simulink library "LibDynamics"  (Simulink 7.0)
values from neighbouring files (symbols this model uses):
  delay = ones(nTbl,1) * mean(valveDelay)    [analysis.m]
  dof = [1 2 3 4 5 6]    [initialize.m]    (also in StaticLiftTransform.m = [3 4 5]; accelEnvelope.m = varargin{1}{1}; displEnvelope.m = varargin{1}{1}; displPivotEnvelope.m = varargin{1}{1})
  flowCanon = 63090.2    [initialize.m]
  forceCanon = 0.00444822    [initialize.m]
  gasConstant = 1.8    [initialize.m]
  gee = geeCanon / linAccelCanon * ~isempty(find(dof==3))    [initialize.m]    (also in accelA2T.m = 0; accelEnvelope.m = varargin{1}{6}; accelT2A.m = 0)
  inertia = inertia + inertiaP2Q([0 0 0], massA(i), cgA(:,i)-cg,  									inertiaCanon, massCanon)    [initialize.m]
  inertiaCanon = 2.9264264e-04    (= 0.00029264264)    [initialize.m]
  initDispl = zeros(6, 1)    [initialize.m]
  lengthCanon = 25.4    [initialize.m]
  linAccelCanon = 9810.0    (= 9810)    [initialize.m]    (also in StaticLiftTransform.m; accelJacobian.m = canon(3); accelP2Q.m = canon(3))
  linDisplCanon = 1    [initialize.m]    (also in StaticLiftTransform.m; displJacobian.m = canon(1))
  linVelocCanon = 1000.0    (= 1000)    [initialize.m]    (also in StaticLiftTransform.m)
  mass = ones(3, 1) * (sum(massA) + massT + massS)    [initialize.m]
  massCanon = 0.4535924e-06    (= 4.535924e-07)    [initialize.m]
  maxDispl = max(abs(maxDispl), abs(minDispl))    [initialize.m]    (also in Tutorial.m = 0.4)
  maxVeloc = max(abs(maxVeloc), abs(minVeloc))    [analysis.m]    (also in initialize.m; rampth.m = 2 * maxDispl / (nVeloc * deltaT); Tutorial.m = 1.234)
  modalCG = [0 0 1000]    [initialize.m]
  modalDamp = [4 5 6]    [initialize.m]    (also in resondemo.m = eval(get(findobj(fig, 'Tag', 'modalDamp'), 'String')))
  modalFreq = [7 6 5]    [initialize.m]    (also in resondemo.m = tableFreq * freqRatio)
  modalMass = 0    [initialize.m]    (also in resondemo.m = tableMass * massRatio)
  oilDamping = 2 * damping * 0.01 * 2 * pi .* oilColumn .* massQ * massCanon    [initialize.m]
  oilSpring = bulkModulus * pressCanon  			.* (area1 * areaCanon ./ length1 + area2 * areaCanon ./ length2)    [initialize.m]
  precharge = 2000    [initialize.m]
  pumpFlow = 1e10    (= 10000000000)    [initialize.m]
  rotAccelCanon = pi/180    (= 0.0174532925199)    [initialize.m]    (also in StaticLiftTransform.m; accelJacobian.m = canon(7); accelP2Q.m = canon(7); bodyAccel.m = canon(3))
  rotDisplCanon = pi/180    (= 0.0174532925199)    [initialize.m]    (also in StaticLiftTransform.m; accelA2T.m = canon(5); accelP2Q.m = canon(5); accelT2A.m = canon(5))
  rotForceCanon = 1000    [initialize.m]    (also in StaticLiftTransform.m)
  rotVelocCanon = pi/180    (= 0.0174532925199)    [initialize.m]    (also in StaticLiftTransform.m; accelJacobian.m = canon(6); accelP2Q.m = canon(6); bodyAccel.m = canon(2))
  samplePeriod = controlPeriod/upsampleFactor    (= 0.00048828125)    [initialize.m]    (also in viewer.m = eval(getHeaderValue(header, 'DELTA_T')))
  supplyPress = 3000    [initialize.m]
  vmax = ( (maxFlow' * flowCanon ./ (area1 * areaCanon)) / linVelocCanon)'    [initialize.m]
  volume = 160    [initialize.m]    (also in quake.m = volume / 231.0)
  volumeCanon = 3785412.0    (= 3785412)    [initialize.m]
undefined symbols (not defined in the file or in its folder): drive, drum, friction, gear, motDisplCanon, motor, motTorqueCanon, motVelocCanon, params, yieldDispl
libraries: LibDynamics x26, LibTransforms x12, aerospace x6, simulink x2
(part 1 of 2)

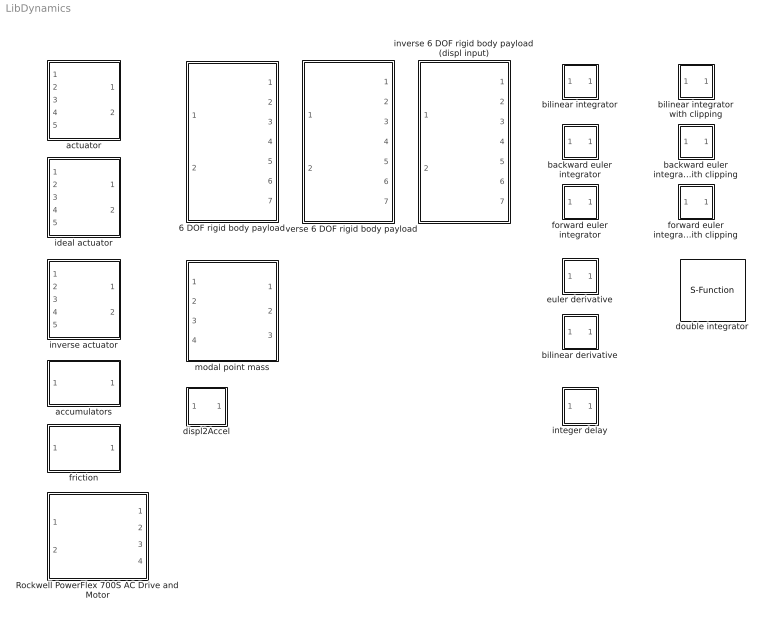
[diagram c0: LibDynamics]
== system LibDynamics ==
  6 DOF rigid body payload : Subsystem  mask(6 DOF Rigid Body Payload Model){mass=mass, inertia=diag(inertia), gee=gee, massCanon=massCanon, inertiaCanon=inertiaCanon, linVelocCanon=linVelocCanon, linAccelCanon=linAccelCanon, rotDisplCanon=rotDisplCanon, rotVelocCanon=rotVelocCanon, rotAccelCanon=rotAccelCanon, rotForceCanon=rotForceCanon, initialPosition=zeros(6,1), samplePeriod=samplePeriod}
      mask prompts: gee "Gravity constant"; massCanon "Canonical mass units"; inertiaCanon "Canonical inertia units"; linVelocCanon "Canonical linear veloc units"; linAccelCanon "Canonical linear accel units"; rotDisplCanon "Canonical rotary displ units"; rotVelocCanon "Canonical rotary veloc units"; rotAccelCanon "Canonical rotary accel units"; rotForceCanon "Canonical rotary force units"; initialPosition "Initial position"; samplePeriod "Sample period (sec)"
      mask init:
      | % invert mass vector
      | invMass = zeros(3,1);
      | nonzero = find(mass>0);
      | invMass(nonzero) = 1 ./ mass(nonzero);
      | 
      | % invert inertia matrix
      | invInertia = zeros(3, 3);
      | nonzero    = find(sum(inertia, 1)>0);
      | invInertia(:,nonzero) = pinv(inertia(nonzero,:));
  Rockwell PowerFlex 700S AC Drive and Motor : Subsystem  mask(Rockwell PowerFlex 700S AC Drive and Motor){MotorNPRPM4=drive.MotorNPRPM4, MotorNPPower5=drive.MotorNPPower5, TotalInertia9=drive.TotalInertia9, SpdTrim3Scale24=drive.SpdTrim3Scale24, InertAccelGain57=drive.InertAccelGain57, SpdRegPGain81=drive.SpdRegPGain81, SpdRegIGain82=drive.SpdRegIGain82, SpdRegAntiBckup84=drive.SpdRegAntiBckup84, SpdErrFiltBW89=drive.SpdErrFiltBW89, SRegFBFiltGain93=drive.SRegFBFiltGain93, SRegFBFiltBW94=drive.SRegFBFiltBW94, NotchAttenuation117=drive.NotchAttenuation117, NotchFiltFreq118=drive.NotchFiltFreq118, TorquePosLimit125=drive.TorquePosLimit125, InertAdaptSel132=drive.InertAdaptSel132, InertAdaptBW133=drive.InertAdaptBW133, InertAdaptGain134=drive.InertAdaptGain134, Stegmann0Cnfg259=drive.Stegmann0Cnfg259, AnlgIn1Scale802=drive.AnlgIn1Scale802, inertia=motor.inertia, canon=[motDisplCanon, motVelocCanon, motTorqueCanon, inertiaCanon], initDispl=initDispl/(motDisplCanon*drum.radius*lengthCanon/gear.ratio), samplePeriod=samplePeriod}
      mask prompts: MotorNPRPM4 "#004: Motor Nameplate Rated Speed (rpm)"; MotorNPPower5 "#005: Motor Nameplate Rated Power (Hp)"; TotalInertia9 "#009:Total Inertia [0.01/2.0/655.0] (sec)"; SpdTrim3Scale24 "#024: Inertia Compensation Aux Gain [-1000.0/1.0/1000.0]"; InertAccelGain57 "#057: Inertia Compensation Gain [0.0/1.0/2.0]"; SpdRegPGain81 "#081: Velocity Proportional Gain [0.0/20.0/600.0]"; SpdRegIGain82 "#082: Velocity Integral Gain [0.0/50.0/100000.0] (1/s)"; SpdRegAntiBckup84 "#084: Velocity Feedforward Gain [0.0 0.0 0.5]"; SpdErrFiltBW89 "#089: Velocity Filter Bandwidth [0.0 200.0 2000.0] (rad/s) (0 disables)"; SRegFBFiltGain93 "#093: Velocity  Feedback Filter Gain [-5.0/1.0/20.0] (>1 lead; <1 lag)"; SRegFBFiltBW94 "#094: Velocity Feedback Filter Bandwidth [0.0/35.0/3760.0] (rad/s)"; NotchAttenuation117 "#117: Notch Attenuation [0/50/500]"; NotchFiltFreq118 "#118: Notch Filter Frequency [0.0/0.0/500.0] (rad/s) (0 disables)"; TorquePosLimit125 "#125: Torque Limit [0.0/2.0/8.0]"; InertAdaptSel132 "#132: Inertia Adaptation Select [0/0/1]"; InertAdaptBW133 "#133: Inertia Adaptation Bandwidth [10.0/100.0/250] (rad/s)"; InertAdaptGain134 "#134: Inertia Adaptation Gain [0.3/0.5/1.0] (use 0 to disable)"; Stegmann0Cnfg259 "#259 Encoder Filter Length Binary Exponent [0/1/7]"; AnlgIn1Scale802 "#802: PU Velocity Per Volt [-2.2e10/0.0/2.2e10] (1/volt)"; inertia "Motor + rigid load inertia"; canon "Canonical units: [displ, veloc, torque, inertia]"; initDispl "Initial displacement"; samplePeriod "Sample period (sec)"
      mask init:
      | % canonical units
      | displCanon	 = canon(1);
      | velocCanon	 = canon(2);
      | torqueCanon	 = canon(3);
      | inertiaCanon = canon(4);
      | 
      | % hardcoded parameters
      | NotchQ		 = 0.67;		% notch filter Q factor
      | StegmannPPR	 = 2^20;		% encoder pulses per revolution
      | 
      | % base quantities for PU system
      | baseTorque	 = MotorNPPower5 * 5252.1 / MotorNPRPM4;	% ft-lb
      | baseSpeed	 = MotorNPRPM4;								% rpm
      | baseDispl	 = baseSpeed/60;							% rev
      | 
      | % disable conditions:  notch filter
      | if (NotchAttenuation117 > 0)
      | 	NotchDepth = -(1 - 1/NotchAttenuation117);
      | else
      | 	NotchDepth = 0;
      | end
      | 
      | % Stegmann encoder filter length
      | filterLength4K	= 2^Stegmann0Cnfg259;				% at 4000 Hz sample rate
      | filterLength1K	= max(1, fix(filterLength4K/4));	% at 1024 Hz sample rate
      | encFilterLength	= filterLength1K;
  accumulators : Subsystem  mask(Accumulator Model){pumpFlow=pumpFlow, supplyPressure=supplyPress, precharge=precharge, bottleVolume=volume, gasConstant=gasConstant, flowCanon=flowCanon, volumeCanon=volumeCanon, samplePeriod=samplePeriod}
      mask prompts: pumpFlow "Pump flow"; supplyPressure "Supply pressure"; precharge "Precharge pressure"; bottleVolume "Bottle volume"; gasConstant "Gas constant"; flowCanon "Canonical flow units"; volumeCanon "Canonical volume units"; samplePeriod "Sample period (sec)"
      mask init:
      | dischargeVolume = bottleVolume * (1 - (precharge/supplyPressure)^(1/gasConstant));
  actuator : Subsystem  mask(Actuator){params=params}
      mask prompts: params "Parameter vector"
  backward euler integrator : Subsystem  mask(Discrete Backward Euler Integrator){initialCondition=0, samplePeriod=samplePeriod}
      mask prompts: initialCondition "Initial condition"; samplePeriod "Sample period (sec)"
  backward euler integrator with clipping : Subsystem  mask(Discrete Backward Euler Integrator with Clipping){initialCondition=0, maxOutput=inf, minOutput=-inf, samplePeriod=samplePeriod}
      mask prompts: initialCondition "Initial condition"; maxOutput "Maximum output"; minOutput "Minimum output"; samplePeriod "Sample period (sec)"
  bilinear derivative : Subsystem  mask(Discrete Bilinear Differentiator){decay=0.9, initialCondition=0, samplePeriod=samplePeriod}
      mask prompts: decay "Decay time constant (0: backward Euler, 1: binlinear)"; initialCondition "Initial condition"; samplePeriod "Sample period"
  bilinear integrator : Subsystem  mask(Discrete Bilinear Integrator){initialCondition=0, samplePeriod=samplePeriod}
      mask prompts: initialCondition "Initial condition"; samplePeriod "Sample period (sec)"
  bilinear integrator with clipping : Subsystem  mask(Discrete Bilinear Integrator with Clipping){initialCondition=0, maxOutput=inf, minOutput=-inf, samplePeriod=samplePeriod}
      mask prompts: initialCondition "Initial condition"; maxOutput "Maximum output"; minOutput "Minimum output"; samplePeriod "Sample period (sec)"
  displ2Accel : Subsystem  mask(Displacement to Body Acceleration Converter){dof=dof, linDisplCanon=linDisplCanon, linAccelCanon=linAccelCanon, rotDisplCanon=rotDisplCanon, rotAccelCanon=rotAccelCanon, freq=40, order=8, samplePeriod=samplePeriod}
      mask prompts: dof "Degree-of-freedom indices"; linDisplCanon "Canonical linear displ units"; linAccelCanon "Canonical linear accel units"; rotDisplCanon "Canonical rotary displ units"; rotAccelCanon "Canonical rotary accel units"; freq "Lowpass filter cutoff freq (Hz)"; order "Lowpass filter order"; samplePeriod "Sample period (sec)"
  double integrator : S-Function  FunctionName=doubleintegrator  Parameters=maxDispl, minDispl, initDispl, maxVeloc, minVeloc, initVeloc, samplePeriod  mask(Double integrator){maxDispl=maxDispl*linDisplCanon, minDispl=-maxDispl*linDisplCanon, initDispl=initDispl*linDisplCanon, maxVeloc=maxVeloc*linVelocCanon, minVeloc=-maxVeloc*linVelocCanon, initVeloc=0, samplePeriod=-1}
      mask prompts: maxDispl "Maximum displacement"; minDispl "Minimum displacement"; initDispl "Initial displacement"; maxVeloc "Maximum velocity"; minVeloc "Minimum velocity"; initVeloc "Initial velocity"; samplePeriod "Sample period (sec)"
      mask help: Integrates acceleration twice to produce velocity and displacement. When clipping occurs, acceleration, velocity and displacement are adjusted accordingly.
  euler derivative : Subsystem  mask(Discrete Euler Derivative){initialCondition=0, samplePeriod=samplePeriod}
      mask prompts: initialCondition "Initial condition"; samplePeriod "Sample period (sec)"
  forward euler integrator : Subsystem  mask(Discrete Forward Euler Integrator){initialCondition=0, samplePeriod=samplePeriod}
      mask prompts: initialCondition "Initial condition"; samplePeriod "Sample period (sec)"
  forward euler integrator with clipping : Subsystem  mask(Discrete Forward Euler Integrator with Clipping){initialCondition=0, maxOutput=inf, minOutput=-inf, samplePeriod=samplePeriod}
      mask prompts: initialCondition "Initial condition"; maxOutput "Maximum output"; minOutput "Minimum output"; samplePeriod "Sample period (sec)"
  friction : Subsystem  mask(Continuous Viscoplastic Friction Law Model){friction=friction * forceCanon, yieldDispl=yieldDispl * lengthCanon, hysteresis=0, velocCanon=linVelocCanon, samplePeriod=samplePeriod}
      mask prompts: friction "Sliding friction"; yieldDispl "Equiv. yield displacement"; hysteresis "Hysteresis constant"; velocCanon "Canonical velocity units"; samplePeriod "Sample period (sec)"
  ideal actuator : Subsystem  mask(Idealized Actuator){kv=vmax * linVelocCanon / 10, spring=oilSpring, damp=oilDamping, delay=0}
      mask prompts: kv "Velocity constant"; spring "Spring constant"; damp "Damping constant"; delay "Servovalve delay"
  integer delay : Subsystem  mask(Integer Delay){initialCondition=0.0, sampleTime=-1, delay=round(delay/samplePeriod)}
      mask prompts: initialCondition "Initial condition"; sampleTime "Sample time"; delay "Number of delays"
      mask help: This delay is the same as Simulink's Integer Delay, with an enhancement that allows a zero delay (which causes an error message from Simulink's delay block).
  inverse 6 DOF rigid body payload : Subsystem  mask(Inverse 6 DOF Rigid Body Payload Model){mass=mass, inertia=diag(inertia), gee=gee, massCanon=massCanon, inertiaCanon=inertiaCanon, linVelocCanon=linVelocCanon, linAccelCanon=linAccelCanon, rotDisplCanon=rotDisplCanon, rotVelocCanon=rotVelocCanon, rotAccelCanon=rotAccelCanon, rotForceCanon=rotForceCanon, initialPosition=zeros(6,1), samplePeriod=samplePeriod}
      mask prompts: gee "Gravity constant"; massCanon "Canonical mass units"; inertiaCanon "Canonical inertia units"; linVelocCanon "Canonical linear veloc units"; linAccelCanon "Canonical linear accel units"; rotDisplCanon "Canonical rotary displ units"; rotVelocCanon "Canonical rotary veloc units"; rotAccelCanon "Canonical rotary accel units"; rotForceCanon "Canonical rotary force units"; initialPosition "Initial position"; samplePeriod "Sample period (sec)"
  inverse 6 DOF rigid body payload (displ input) : Subsystem  mask(Inverse 6 DOF Rigid Body Payload Model (Displacement Input)){mass=mass, inertia=diag(inertia), gee=gee, massCanon=massCanon, inertiaCanon=inertiaCanon, linVelocCanon=linVelocCanon, linAccelCanon=linAccelCanon, rotDisplCanon=rotDisplCanon, rotVelocCanon=rotVelocCanon, rotAccelCanon=rotAccelCanon, rotForceCanon=rotForceCanon, initialPosition=zeros(6,1), samplePeriod=samplePeriod}
      mask prompts: gee "Gravity constant"; massCanon "Canonical mass units"; inertiaCanon "Canonical inertia units"; linVelocCanon "Canonical linear veloc units"; linAccelCanon "Canonical linear accel units"; rotDisplCanon "Canonical rotary displ units"; rotVelocCanon "Canonical rotary veloc units"; rotAccelCanon "Canonical rotary accel units"; rotForceCanon "Canonical rotary force units"; initialPosition "Initial position"; samplePeriod "Sample period (sec)"
  inverse actuator : Subsystem  mask(Inverse actuator){params=params}
      mask prompts: params "Parameter vector"
  modal point mass : Subsystem  mask(Modal Point Mass){mass=modalMass, freq=modalFreq, damp=modalDamp, ofst=modalCG, gee=gee, massCanon=massCanon, linAccelCanon=linAccelCanon, rotDisplCanon=rotDisplCanon, rotVelocCanon=rotVelocCanon, rotForceCanon=rotForceCanon, samplePeriod=samplePeriod}
      mask prompts: freq "Natural frequency (Hz)"; damp "Damping (percent)"; ofst "Offset from origin"; gee "Gravity constant"; massCanon "Canonical mass units"; linAccelCanon "Canonical linear accel units"; rotDisplCanon "Canonical rotary displ units"; rotVelocCanon "Canonical rotary veloc units"; rotForceCanon "Canonical rotary force units"; samplePeriod "Sample period (sec)"
      mask init:
      | a = zeros(3,3);
      | b = zeros(3,3);
      | for i = 1:3		% for x, y, z
      | 	if (0 < freq(i)) & (freq(i) * samplePeriod < 0.5) & (mass > 0)
      | 		as = [1 2*0.01*damp(i)*2*pi*freq(i) (2*pi*freq(i)).^2];
      | 		bs = as(2:3);
      | 		[b(i,:), a(i,:)] = bilinear(bs, as, 1/samplePeriod);
      | 	else
      | 		b(i,:) = [0 0 0];
      | 		a(i,:) = [1 0 0];
      | 	end
      | end

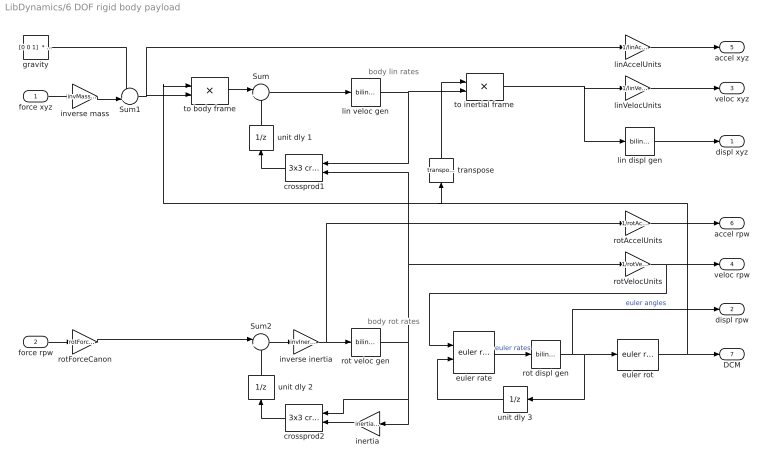
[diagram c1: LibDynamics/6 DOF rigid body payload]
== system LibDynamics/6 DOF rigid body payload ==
  note: body rot rates
  note: body lin rates
  force xyz : Inport  OutDataType=sfix(16)  OutScaling=2^0
  force rpw : Inport  Port=2  OutDataType=sfix(16)  OutScaling=2^0
  Sum : Sum  Inputs=|++  OutDataType=sfix(16)  OutScaling=2^0
  Sum1 : Sum  Inputs=-+|  OutDataType=sfix(16)  OutScaling=2^0
  Sum2 : Sum  Inputs=|+-  OutDataType=sfix(16)  OutScaling=2^0
  crossprod1 : aerospace/Axes Transformations/3x3 cross product  Orientation=left  SystemSampleTime=-1
  crossprod2 : aerospace/Axes Transformations/3x3 cross product  Orientation=left  SystemSampleTime=-1
  euler rate : LibTransforms/euler rate  SystemSampleTime=-1
  euler rot : LibTransforms/euler rot  SystemSampleTime=-1
  gravity : Constant  Value="[0 0 1]  * gee *  linAccelCanon"  OutDataType=sfix(16)  OutScaling=2^0
  inertia : Gain  Orientation=left  Gain=inertia*inertiaCanon  Multiplication=Matrix(K*u)  ParameterDataType=sfix(16)  ParameterScaling=2^0  OutDataType=sfix(16)  OutScaling=2^0
  inverse inertia : Gain  Gain=invInertia/inertiaCanon  Multiplication=Matrix(K*u)  ParameterDataType=sfix(16)  ParameterScaling=2^0  OutDataType=sfix(16)  OutScaling=2^0
  inverse mass : Gain  Gain=invMass/massCanon  ParameterDataType=sfix(16)  ParameterScaling=2^0  OutDataType=sfix(16)  OutScaling=2^0
  lin displ gen : LibDynamics/bilinear integrator  SystemSampleTime=-1  initialCondition=initialPosition(1:3)  samplePeriod=samplePeriod
  lin veloc gen : LibDynamics/bilinear integrator  SystemSampleTime=-1  initialCondition=0  samplePeriod=samplePeriod
  linAccelUnits : Gain  Gain=1/linAccelCanon  ParameterDataType=sfix(16)  ParameterScaling=2^0  OutDataType=sfix(16)  OutScaling=2^0
  linVelocUnits : Gain  Gain=1/linVelocCanon  ParameterDataType=sfix(16)  ParameterScaling=2^0  OutDataType=sfix(16)  OutScaling=2^0
  rot displ gen : LibDynamics/bilinear integrator  SystemSampleTime=-1  initialCondition=initialPosition(4:6)  samplePeriod=samplePeriod
  rot veloc gen : LibDynamics/bilinear integrator  SystemSampleTime=-1  initialCondition=0  samplePeriod=samplePeriod
  rotAccelUnits : Gain  Gain=1/rotAccelCanon  ParameterDataType=sfix(16)  ParameterScaling=2^0  OutDataType=sfix(16)  OutScaling=2^0
  rotForceCanon : Gain  Gain=rotForceCanon  ParameterDataType=sfix(16)  ParameterScaling=2^0  OutDataType=sfix(16)  OutScaling=2^0
  rotVelocUnits : Gain  Gain=1/rotVelocCanon  ParameterDataType=sfix(16)  ParameterScaling=2^0  OutDataType=sfix(16)  OutScaling=2^0
  to body frame : Product  Multiplication=Matrix(*)  OutDataType=sfix(16)  OutScaling=2^0
  to inertial frame : Product  Multiplication=Matrix(*)  OutDataType=sfix(16)  OutScaling=2^0
  transpose : Math  Orientation=up  Operator=transpose  OutDataType=sfix(16)  OutScaling=2^0
  unit dly 1 : UnitDelay  Orientation=up  SampleTime=-1
  unit dly 2 : UnitDelay  Orientation=up  SampleTime=-1
  unit dly 3 : UnitDelay  Orientation=left  X0=initialPosition(4:6)  SampleTime=-1
  displ xyz : Outport  OutDataType=sfix(16)  OutScaling=2^0
  displ rpw : Outport  Port=2  OutDataType=sfix(16)  OutScaling=2^0
  veloc xyz : Outport  Port=3  OutDataType=sfix(16)  OutScaling=2^0
  veloc rpw : Outport  Port=4  OutDataType=sfix(16)  OutScaling=2^0
  accel xyz : Outport  Port=5  OutDataType=sfix(16)  OutScaling=2^0
  accel rpw : Outport  Port=6  OutDataType=sfix(16)  OutScaling=2^0
  DCM : Outport  Port=7  OutDataType=sfix(16)  OutScaling=2^0
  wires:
  to body frame/1 -> Sum/1
  Sum1/1 -> linAccelUnits/1, to body frame/2
  inverse mass/1 -> Sum1/2
  force xyz/1 -> inverse mass/1
  gravity/1 -> Sum1/1
  crossprod1/1 -> unit dly 1/1
  transpose/1 -> to inertial frame/1
  to inertial frame/1 -> linVelocUnits/1, lin displ gen/1
  linVelocUnits/1 -> veloc xyz/1
  inertia/1 -> crossprod2/2
  rotForceCanon/1 -> Sum2/1
  inverse inertia/1 -> rotAccelUnits/1, rot veloc gen/1
  Sum2/1 -> inverse inertia/1
  rotAccelUnits/1 -> accel rpw/1
  rotVelocUnits/1 -> veloc rpw/1, euler rate/1
  rot displ gen/1 -> displ rpw/1, unit dly 3/1, euler rot/1  "euler angles"
  crossprod2/1 -> unit dly 2/1
  Sum/1 -> lin veloc gen/1
  lin displ gen/1 -> displ xyz/1
  linAccelUnits/1 -> accel xyz/1
  euler rot/1 -> DCM/1, transpose/1, to body frame/1
  euler rate/1 -> rot displ gen/1  "euler rates"
  force rpw/1 -> rotForceCanon/1
  lin veloc gen/1 -> crossprod1/1, to inertial frame/2
  rot veloc gen/1 -> inertia/1, crossprod2/1, rotVelocUnits/1, crossprod1/2
  unit dly 1/1 -> Sum/2
  unit dly 2/1 -> Sum2/2
  unit dly 3/1 -> euler rate/2

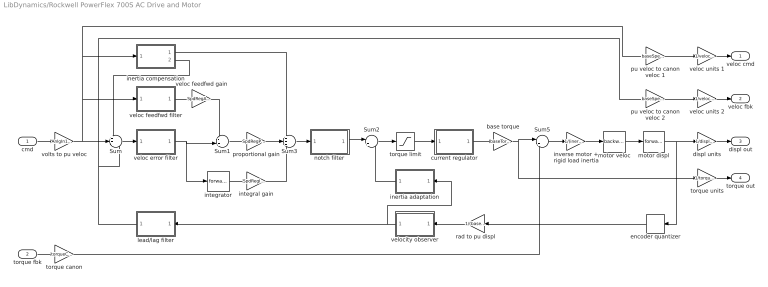
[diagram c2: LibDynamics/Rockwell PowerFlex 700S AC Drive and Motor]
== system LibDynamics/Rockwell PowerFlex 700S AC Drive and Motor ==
  cmd : Inport  OutDataType=sfix(16)  OutScaling=2^0
  torque fbk : Inport  Port=2  OutDataType=sfix(16)  OutScaling=2^0
  Sum : Sum  Inputs=++-  OutDataType=sfix(16)  OutScaling=2^0
  Sum1 : Sum  Inputs=-+|  OutDataType=sfix(16)  OutScaling=2^0
  Sum2 : Sum  Inputs=|+-  OutDataType=sfix(16)  OutScaling=2^0
  Sum3 : Sum  Inputs=+++  OutDataType=sfix(16)  OutScaling=2^0
  Sum5 : Sum  Inputs=|+-  OutDataType=sfix(16)  OutScaling=2^0
  base torque : Gain  Gain=baseTorque*torqueCanon  ParameterDataType=sfix(16)  ParameterScaling=2^0  OutDataType=sfix(16)  OutScaling=2^0
  current regulator : Subsystem
  displ units : Gain  Gain=1/displCanon  ParameterDataType=sfix(16)  ParameterScaling=2^0  OutDataType=sfix(16)  OutScaling=2^0
  encoder quantizer : Quantizer  Orientation=left  QuantizationInterval=2*pi/StegmannPPR
  inertia adaptation : Subsystem  Orientation=left
  inertia compensation : Subsystem
  integral gain : Gain  Gain=SpdRegIGain82  ParameterDataType=sfix(16)  ParameterScaling=2^0  OutDataType=sfix(16)  OutScaling=2^0
  integrator : LibDynamics/forward euler integrator  SystemSampleTime=-1  initialCondition=0  samplePeriod=samplePeriod
  inverse motor + rigid load inertia : Gain  Gain=1/(inertia*inertiaCanon)  ParameterDataType=sfix(16)  ParameterScaling=2^0  OutDataType=sfix(16)  OutScaling=2^0
  lead/lag filter : Subsystem  Orientation=left  mask(Discrete-Time Approximation to Continuous-Time Lead-Lag Filter){k=SRegFBFiltGain93, w=SRegFBFiltBW94, period=samplePeriod}
      mask prompts: k "Gain"; w "Frequency (rad/s)"; period "Sample period (sec)"
      mask init:
      | if w > 0
      | 	bs = [k w];
      | 	as = [1 w];
      | 	[b a] = bilinear(bs, as, 1/period);
      | else
      | 	b  = [1];
      | 	a  = [1];
      | end
  motor displ : LibDynamics/forward euler integrator  SystemSampleTime=-1  initialCondition=initDispl * displCanon  samplePeriod=samplePeriod
  motor veloc : LibDynamics/backward euler integrator  SystemSampleTime=-1  initialCondition=0  samplePeriod=samplePeriod
  notch filter : Subsystem  mask{freq=NotchFiltFreq118/(2*pi), bw=(NotchFiltFreq118/(2*pi))/NotchQ, depth=NotchDepth, gain=1, period=samplePeriod}
      mask prompts: freq "Center frequency (Hz)"; bw "3 dB bandwidth (Hz)"; depth "Notch depth"; gain "DC gain"; period "Sample period (sec)"
      mask init:
      | if (0 < freq) & (freq * period < 0.5)
      | 	t	 = tan(pi * bw * period);	
      | 	k1	 = -cos(2 * pi * freq * period);
      | 	k1	 = max(min(k1, 1), -1);
      | 	k2	 = (1.0 - t) / (1.0 + t);
      | 	k2	 = max(min(k2, 1), -1);
      | 	w0	 =  gain + 0.5 * depth;
      | 	w1	 = -0.5 * depth;
      | else
      | 	k1	 = 0.0;
      | 	k2	 = 0.0;
      | 	w0	 = gain;
      | 	w1	 = 0.0;
      | end
      | a1	= k1 * (1 + k2);
      | a2	= k2;
      | b	= [w0+w1*a2 (w0+w1)*a1 w1+w0*a2];
      | a	= [1 a1 a2];
  proportional gain : Gain  Gain=SpdRegPGain81  ParameterDataType=sfix(16)  ParameterScaling=2^0  OutDataType=sfix(16)  OutScaling=2^0
  pu veloc to canon veloc 1 : Gain  Gain=baseSpeed*velocCanon  ParameterDataType=sfix(16)  ParameterScaling=2^0  OutDataType=sfix(16)  OutScaling=2^0
  pu veloc to canon veloc 2 : Gain  Gain=baseSpeed*velocCanon  ParameterDataType=sfix(16)  ParameterScaling=2^0  OutDataType=sfix(16)  OutScaling=2^0
  rad to pu displ : Gain  Orientation=left  Gain=1/(baseSpeed*velocCanon)  ParameterDataType=sfix(16)  ParameterScaling=2^0  OutDataType=sfix(16)  OutScaling=2^0
  torque limit : Saturate  UpperLimit=TorquePosLimit125  LowerLimit=-TorquePosLimit125
  torque canon : Gain  Gain=torqueCanon  ParameterDataType=sfix(16)  ParameterScaling=2^0  OutDataType=sfix(16)  OutScaling=2^0
  torque units : Gain  Gain=1/torqueCanon  ParameterDataType=sfix(16)  ParameterScaling=2^0  OutDataType=sfix(16)  OutScaling=2^0
  veloc feedfwd gain : Gain  Gain=SpdRegAntiBckup84  ParameterDataType=sfix(16)  ParameterScaling=2^0  OutDataType=sfix(16)  OutScaling=2^0
  veloc error filter : Subsystem  mask(Velocity filter){bw=SpdErrFiltBW89, period=samplePeriod}
      mask prompts: bw "Bandwidth (rad/s)"; period "Sample period (sec)"
      mask init:
      | if bw > 0
      | 	bs	= [bw^2];
      | 	as	= [1 2*bw bw^2];
      | 	[b a] = impinvar(bs, as, 1/period);
      | 	b	= b(2:end);				% lop off leading zero
      | 	b	= b * sum(a)/sum(b);	% adjust dc gain
      | else
      | 	b = [1];
      | 	a = [1];
      | end
  veloc feedfwd filter : Subsystem  mask(Velocity filter){bw=SpdErrFiltBW89, period=samplePeriod}
      mask prompts: bw "Bandwidth (rad/s)"; period "Sample period (sec)"
      mask init:
      | if bw > 0
      | 	bs	= [bw^2];
      | 	as	= [1 2*bw bw^2];
      | 	[b a] = impinvar(bs, as, 1/period);
      | 	b	= b(2:end);				% lop off leading zero
      | 	b	= b * sum(a)/sum(b);	% adjust dc gain
      | else
      | 	b = [1];
      | 	a = [1];
      | end
  veloc units 1 : Gain  Gain=1/velocCanon  ParameterDataType=sfix(16)  ParameterScaling=2^0  OutDataType=sfix(16)  OutScaling=2^0
  veloc units 2 : Gain  Gain=1/velocCanon  ParameterDataType=sfix(16)  ParameterScaling=2^0  OutDataType=sfix(16)  OutScaling=2^0
  velocity observer : Subsystem  Orientation=left
  volts to pu veloc : Gain  Gain=AnlgIn1Scale802  ParameterDataType=sfix(16)  ParameterScaling=2^0  OutDataType=sfix(16)  OutScaling=2^0
  veloc cmd : Outport  OutDataType=sfix(16)  OutScaling=2^0
  veloc fbk : Outport  Port=2  OutDataType=sfix(16)  OutScaling=2^0
  displ out : Outport  Port=3  OutDataType=sfix(16)  OutScaling=2^0
  torque out : Outport  Port=4  OutDataType=sfix(16)  OutScaling=2^0
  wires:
  inertia compensation/2(aux) -> Sum/1
  volts to pu veloc/1 -> Sum/2, pu veloc to canon veloc 1/1, inertia compensation/1(inp), veloc feedfwd filter/1(inp)
  Sum/1 -> veloc error filter/1(inp)
  veloc error filter/1(out) -> Sum1/2, integrator/1
  Sum1/1 -> proportional gain/1
  integrator/1 -> integral gain/1
  velocity observer/1(out) -> lead/lag filter/1(inp), inertia adaptation/1(inp)
  lead/lag filter/1(out) -> Sum/3, pu veloc to canon veloc 2/1
  torque limit/1 -> current regulator/1(inp)
  Sum5/1 -> inverse motor + rigid load inertia/1
  veloc feedfwd filter/1(out) -> veloc feedfwd gain/1
  current regulator/1(out) -> base torque/1
  torque fbk/1 -> torque canon/1
  cmd/1 -> volts to pu veloc/1
  base torque/1 -> Sum5/1, torque units/1
  encoder quantizer/1 -> rad to pu displ/1
  veloc feedfwd gain/1 -> Sum1/1
  proportional gain/1 -> Sum3/2
  integral gain/1 -> Sum3/3
  inertia compensation/1(out) -> Sum3/1
  Sum3/1 -> notch filter/1(inp)
  notch filter/1(out) -> Sum2/1
  Sum2/1 -> torque limit/1
  inertia adaptation/1(out) -> Sum2/2
  pu veloc to canon veloc 1/1 -> veloc units 1/1
  veloc units 1/1 -> veloc cmd/1
  torque units/1 -> torque out/1
  displ units/1 -> displ out/1
  inverse motor + rigid load inertia/1 -> motor veloc/1
  motor veloc/1 -> motor displ/1
  motor displ/1 -> displ units/1, encoder quantizer/1
  veloc units 2/1 -> veloc fbk/1
  torque canon/1 -> Sum5/2
  rad to pu displ/1 -> velocity observer/1(inp)
  pu veloc to canon veloc 2/1 -> veloc units 2/1

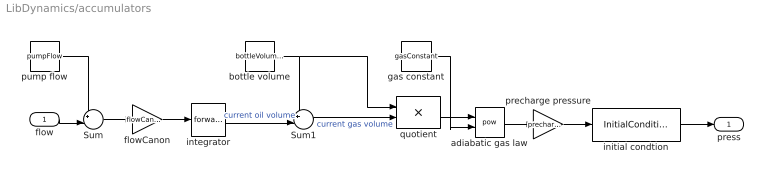
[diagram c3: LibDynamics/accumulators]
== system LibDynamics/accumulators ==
  flow : Inport  OutDataType=sfix(16)  OutScaling=2^0
  Sum : Sum  Inputs=+-|  OutDataType=sfix(16)  OutScaling=2^0
  Sum1 : Sum  Inputs=+-|  OutDataType=sfix(16)  OutScaling=2^0
  adiabatic gas law : Math  Operator=pow  OutDataType=sfix(16)  OutScaling=2^0
  bottle volume : Constant  Value=bottleVolume*volumeCanon  OutDataType=sfix(16)  OutScaling=2^0
  flowCanon : Gain  Gain=flowCanon  ParameterDataType=sfix(16)  ParameterScaling=2^0  OutDataType=sfix(16)  OutScaling=2^0
  gas constant : Constant  Value=gasConstant  OutDataType=sfix(16)  OutScaling=2^0
  initial condtion : InitialCondition  Value=supplyPressure
  integrator : LibDynamics/forward euler integrator with clipping  SystemSampleTime=-1  initialCondition=dischargeVolume*volumeCanon  maxOutput=dischargeVolume*volumeCanon  minOutput=0  samplePeriod=samplePeriod
  precharge pressure : Gain  Gain=precharge  ParameterDataType=sfix(16)  ParameterScaling=2^0  OutDataType=sfix(16)  OutScaling=2^0
  pump flow : Constant  Value=pumpFlow  OutDataType=sfix(16)  OutScaling=2^0
  quotient : Product  Inputs=*/  OutDataType=sfix(16)  OutScaling=2^0
  press : Outport  OutDataType=sfix(16)  OutScaling=2^0
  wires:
  pump flow/1 -> Sum/1
  Sum/1 -> flowCanon/1
  bottle volume/1 -> Sum1/1, quotient/1
  gas constant/1 -> adiabatic gas law/2
  adiabatic gas law/1 -> precharge pressure/1
  precharge pressure/1 -> initial condtion/1
  Sum1/1 -> quotient/2  "current gas volume"
  quotient/1 -> adiabatic gas law/1
  integrator/1 -> Sum1/2  "current oil volume"
  flow/1 -> Sum/2
  flowCanon/1 -> integrator/1
  initial condtion/1 -> press/1

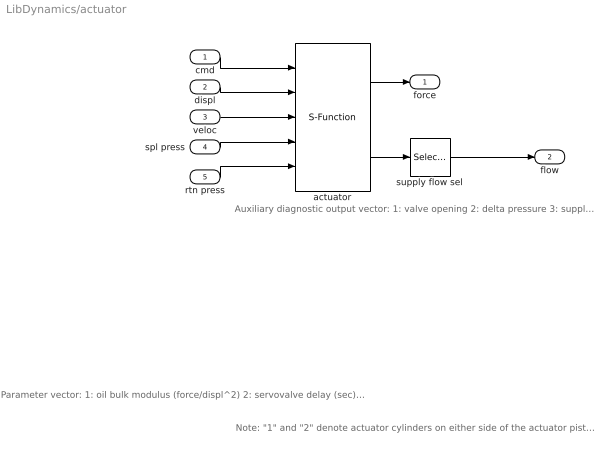
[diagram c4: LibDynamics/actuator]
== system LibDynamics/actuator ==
  note: Auxiliary diagnostic output vector: 1: valve opening 2: delta pressure 3: supply flow 4: return flow 5: C1 pressure 6: C2 pressure 7: C1 flow 8: C2 flow 9: C1 oilspring displacement 10: C2 oilspring displacement 11: C1 oilspring velocity 12: C2 oilspring velocity
  note: Note: "1" and "2" denote actuator cylinders on either side of the actuator piston. With positive valve drive, oil is ported into cylinder 1, resulting in positive displacement.
  note: Parameter vector: 1: oil bulk modulus (force/displ^2) 2: servovalve delay (sec) 3: servovalve overlap 4: rated pressure (force/displ^2) 5: rated flow at rated pressure (displ^3/sec) 6: nominal flow at rated pressure (displ^3/sec) 7: actuator piston area 1 (displ^2) 8: actuator piston area 2 (displ^2) 9: actuator usable stroke 1 (displ) 10: actuator usable stroke 2 (displ) 11: actuator end cushion length 1 (displ) 12: actuator end cushion length 2 (displ) 13: additional port volume 1 (displ^3) 14: additional port volume 2 (displ^3) 15: actuator parasitic damping factor 16: cross-chamber leakage factor (flow/press) 17: ratio port openings according to area 18: sample period (sec) Conversion factors used for converting signals from external (user) to internal (canonical) units: 19: displacement 20: velocity 21: force 22: pressure 23: flow
  cmd : Inport  OutDataType=sfix(16)  OutScaling=2^0
  displ : Inport  Port=2  OutDataType=sfix(16)  OutScaling=2^0
  veloc : Inport  Port=3  OutDataType=sfix(16)  OutScaling=2^0
  spl press : Inport  Port=4  OutDataType=sfix(16)  OutScaling=2^0
  rtn press : Inport  Port=5  OutDataType=sfix(16)  OutScaling=2^0
  actuator : S-Function  FunctionName=Actuator  Parameters=params
  supply flow sel : Selector  IndexOptions=Index vector (dialog)  Indices=3  OutputSizes=1
  force : Outport  OutDataType=sfix(16)  OutScaling=2^0
  flow : Outport  Port=2  OutDataType=sfix(16)  OutScaling=2^0
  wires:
  spl press/1 -> actuator/4
  rtn press/1 -> actuator/5
  cmd/1 -> actuator/1
  actuator/1 -> force/1
  displ/1 -> actuator/2
  veloc/1 -> actuator/3
  actuator/2 -> supply flow sel/1
  supply flow sel/1 -> flow/1

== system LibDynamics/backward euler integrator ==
  inp : Inport  OutDataType=sfix(16)  OutScaling=2^0
  Sum1 : Sum  Inputs=|++  OutDataType=sfix(16)  OutScaling=2^0
  T : Gain  Gain=samplePeriod  ParameterDataType=sfix(16)  ParameterScaling=2^0  OutDataType=sfix(16)  OutScaling=2^0
  Unit Delay1 : UnitDelay  Orientation=left  X0=initialCondition  SampleTime=-1
  out : Outport  OutDataType=sfix(16)  OutScaling=2^0
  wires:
  inp/1 -> T/1
  Unit Delay1/1 -> Sum1/2
  Sum1/1 -> Unit Delay1/1, out/1
  T/1 -> Sum1/1

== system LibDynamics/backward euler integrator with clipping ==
  inp : Inport  OutDataType=sfix(16)  OutScaling=2^0
  Saturation : Saturate  UpperLimit=maxOutput  LowerLimit=minOutput
  Sum1 : Sum  Inputs=|++  OutDataType=sfix(16)  OutScaling=2^0
  T : Gain  Gain=samplePeriod  ParameterDataType=sfix(16)  ParameterScaling=2^0  OutDataType=sfix(16)  OutScaling=2^0
  Unit Delay1 : UnitDelay  Orientation=left  X0=initialCondition  SampleTime=-1
  out : Outport  OutDataType=sfix(16)  OutScaling=2^0
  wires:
  T/1 -> Sum1/1
  Sum1/1 -> Saturation/1
  Unit Delay1/1 -> Sum1/2
  inp/1 -> T/1
  Saturation/1 -> out/1, Unit Delay1/1

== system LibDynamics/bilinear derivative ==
  inp : Inport  OutDataType=sfix(16)  OutScaling=2^0
  (1+decay)/T : Gain  Gain=(1+decay)/samplePeriod  ParameterDataType=sfix(16)  ParameterScaling=2^0  OutDataType=sfix(16)  OutScaling=2^0
  -decay : Gain  Orientation=left  Gain=-decay  ParameterDataType=sfix(16)  ParameterScaling=2^0  OutDataType=sfix(16)  OutScaling=2^0
  Sum : Sum  Inputs=|+-  OutDataType=sfix(16)  OutScaling=2^0
  Sum1 : Sum  Inputs=|++  OutDataType=sfix(16)  OutScaling=2^0
  Unit Delay : UnitDelay  X0=initialCondition  SampleTime=-1
  Unit Delay1 : UnitDelay  Orientation=left  SampleTime=-1
  out : Outport  OutDataType=sfix(16)  OutScaling=2^0
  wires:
  (1+decay)/T/1 -> Sum1/1
  Sum1/1 -> Unit Delay1/1, out/1
  -decay/1 -> Sum1/2
  Unit Delay/1 -> Sum/2
  inp/1 -> Unit Delay/1, Sum/1
  Unit Delay1/1 -> -decay/1
  Sum/1 -> (1+decay)/T/1

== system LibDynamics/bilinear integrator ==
  inp : Inport  OutDataType=sfix(16)  OutScaling=2^0
  Sum : Sum  Inputs=|++  OutDataType=sfix(16)  OutScaling=2^0
  Sum1 : Sum  Inputs=|++  OutDataType=sfix(16)  OutScaling=2^0
  T/2 : Gain  Gain=samplePeriod/2  ParameterDataType=sfix(16)  ParameterScaling=2^0  OutDataType=sfix(16)  OutScaling=2^0
  Unit Delay : UnitDelay  SampleTime=-1
  Unit Delay1 : UnitDelay  Orientation=left  X0=initialCondition  SampleTime=-1
  out : Outport  OutDataType=sfix(16)  OutScaling=2^0
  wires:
  T/2/1 -> Sum1/1
  Sum1/1 -> out/1, Unit Delay1/1
  Unit Delay1/1 -> Sum1/2
  Unit Delay/1 -> Sum/2
  inp/1 -> Sum/1, Unit Delay/1
  Sum/1 -> T/2/1

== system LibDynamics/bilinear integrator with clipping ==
  inp : Inport  OutDataType=sfix(16)  OutScaling=2^0
  Saturation : Saturate  UpperLimit=maxOutput  LowerLimit=minOutput
  Sum : Sum  Inputs=|++  OutDataType=sfix(16)  OutScaling=2^0
  Sum1 : Sum  Inputs=|++  OutDataType=sfix(16)  OutScaling=2^0
  T/2 : Gain  Gain=samplePeriod/2  ParameterDataType=sfix(16)  ParameterScaling=2^0  OutDataType=sfix(16)  OutScaling=2^0
  Unit Delay : UnitDelay  SampleTime=-1
  Unit Delay1 : UnitDelay  Orientation=left  X0=initialCondition  SampleTime=-1
  out : Outport  OutDataType=sfix(16)  OutScaling=2^0
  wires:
  Sum/1 -> T/2/1
  inp/1 -> Unit Delay/1, Sum/1
  Unit Delay/1 -> Sum/2
  Unit Delay1/1 -> Sum1/2
  Sum1/1 -> Saturation/1
  T/2/1 -> Sum1/1
  Saturation/1 -> Unit Delay1/1, out/1

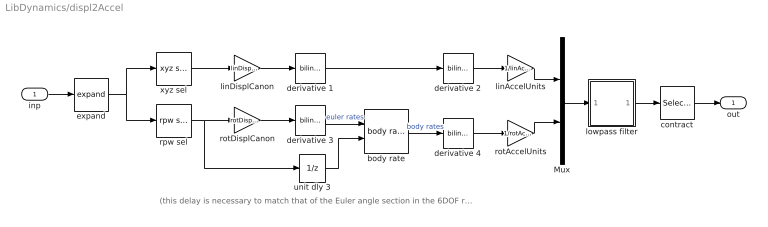
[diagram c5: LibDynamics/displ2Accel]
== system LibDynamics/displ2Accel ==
  note: (this delay is necessary to match that of the Euler angle section in the 6DOF rigid body model)
  inp : Inport  OutDataType=sfix(16)  OutScaling=2^0
  Mux : Mux  Inputs=2
  body rate : LibTransforms/body rate  SystemSampleTime=-1
  contract : Selector  IndexOptions=Index vector (dialog)  Indices=dof  OutputSizes=1
  derivative {1..4} (4 alike) : LibDynamics/bilinear derivative  SystemSampleTime=-1  decay=0.9  samplePeriod=samplePeriod
  expand : LibTransforms/expand  SystemSampleTime=-1  size=6  elements=dof
  linAccelUnits : Gain  Gain=1/linAccelCanon  ParameterDataType=sfix(16)  ParameterScaling=2^0  OutDataType=sfix(16)  OutScaling=2^0
  linDisplCanon : Gain  Gain=linDisplCanon  ParameterDataType=sfix(16)  ParameterScaling=2^0  OutDataType=sfix(16)  OutScaling=2^0
  lowpass filter : Subsystem  mask(6-Channel Butterworth Lowpass Filter){freq=freq, order=order, samplePeriod=samplePeriod}
      mask prompts: freq "Cutoff frequency (Hz)"; order "Filter order"; samplePeriod "Sample period (sec)"
  rotAccelUnits : Gain  Gain=1/rotAccelCanon  ParameterDataType=sfix(16)  ParameterScaling=2^0  OutDataType=sfix(16)  OutScaling=2^0
  rotDisplCanon : Gain  Gain=rotDisplCanon  ParameterDataType=sfix(16)  ParameterScaling=2^0  OutDataType=sfix(16)  OutScaling=2^0
  rpw sel : LibTransforms/rpw sel  SystemSampleTime=-1  dof=1:6
  unit dly 3 : UnitDelay  SampleTime=-1
  xyz sel : LibTransforms/xyz sel  SystemSampleTime=-1  dof=1:6
  out : Outport  OutDataType=sfix(16)  OutScaling=2^0
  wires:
  contract/1 -> out/1
  expand/1 -> xyz sel/1, rpw sel/1
  rotAccelUnits/1 -> Mux/2
  rotDisplCanon/1 -> derivative 3/1
  lowpass filter/1(out) -> contract/1
  derivative 4/1 -> rotAccelUnits/1
  derivative 2/1 -> linAccelUnits/1
  Mux/1 -> lowpass filter/1(inp)
  linAccelUnits/1 -> Mux/1
  xyz sel/1 -> linDisplCanon/1
  rpw sel/1 -> rotDisplCanon/1, unit dly 3/1
  inp/1 -> expand/1
  derivative 1/1 -> derivative 2/1
  linDisplCanon/1 -> derivative 1/1
  derivative 3/1 -> body rate/1  "euler rates"
  body rate/1 -> derivative 4/1  "body rates"
  unit dly 3/1 -> body rate/2

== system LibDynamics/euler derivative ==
  inp : Inport  OutDataType=sfix(16)  OutScaling=2^0
  1/T : Gain  Gain=1/samplePeriod  ParameterDataType=sfix(16)  ParameterScaling=2^0  OutDataType=sfix(16)  OutScaling=2^0
  Sum : Sum  Inputs=|+-  OutDataType=sfix(16)  OutScaling=2^0
  Unit Delay : UnitDelay  X0=initialCondition  SampleTime=-1
  out : Outport  OutDataType=sfix(16)  OutScaling=2^0
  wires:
  1/T/1 -> out/1
  Unit Delay/1 -> Sum/2
  inp/1 -> Sum/1, Unit Delay/1
  Sum/1 -> 1/T/1

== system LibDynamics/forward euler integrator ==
  inp : Inport  OutDataType=sfix(16)  OutScaling=2^0
  Sum1 : Sum  Inputs=|++  OutDataType=sfix(16)  OutScaling=2^0
  T : Gain  Gain=samplePeriod  ParameterDataType=sfix(16)  ParameterScaling=2^0  OutDataType=sfix(16)  OutScaling=2^0
  Unit Delay : UnitDelay  SampleTime=-1
  Unit Delay1 : UnitDelay  Orientation=left  X0=initialCondition  SampleTime=-1
  out : Outport  OutDataType=sfix(16)  OutScaling=2^0
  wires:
  inp/1 -> Unit Delay/1
  Unit Delay/1 -> T/1
  Unit Delay1/1 -> Sum1/2
  Sum1/1 -> Unit Delay1/1, out/1
  T/1 -> Sum1/1

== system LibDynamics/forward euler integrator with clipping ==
  inp : Inport  OutDataType=sfix(16)  OutScaling=2^0
  Saturation : Saturate  UpperLimit=maxOutput  LowerLimit=minOutput
  Sum1 : Sum  Inputs=|++  OutDataType=sfix(16)  OutScaling=2^0
  T : Gain  Gain=samplePeriod  ParameterDataType=sfix(16)  ParameterScaling=2^0  OutDataType=sfix(16)  OutScaling=2^0
  Unit Delay : UnitDelay  SampleTime=-1
  Unit Delay1 : UnitDelay  Orientation=left  X0=initialCondition  SampleTime=-1
  out : Outport  OutDataType=sfix(16)  OutScaling=2^0
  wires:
  T/1 -> Sum1/1
  Sum1/1 -> Saturation/1
  Unit Delay1/1 -> Sum1/2
  Unit Delay/1 -> T/1
  inp/1 -> Unit Delay/1
  Saturation/1 -> out/1, Unit Delay1/1

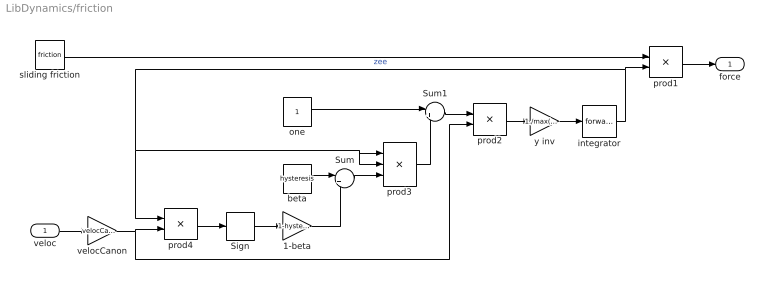
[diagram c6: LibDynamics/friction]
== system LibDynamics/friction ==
  veloc : Inport  OutDataType=sfix(16)  OutScaling=2^0
  1-beta : Gain  Gain=1-hysteresis  ParameterDataType=sfix(16)  ParameterScaling=2^0  OutDataType=sfix(16)  OutScaling=2^0
  Sign : Signum
  Sum : Sum  Inputs=|++  OutDataType=sfix(16)  OutScaling=2^0
  Sum1 : Sum  Inputs=|+-  OutDataType=sfix(16)  OutScaling=2^0
  beta : Constant  Value=hysteresis  OutDataType=sfix(16)  OutScaling=2^0
  integrator : LibDynamics/forward euler integrator with clipping  SystemSampleTime=-1  initialCondition=0  maxOutput=1  minOutput=-1  samplePeriod=samplePeriod
  one : Constant  OutDataType=sfix(16)  OutScaling=2^0
  prod1 : Product  OutDataType=sfix(16)  OutScaling=2^0
  prod2 : Product  OutDataType=sfix(16)  OutScaling=2^0
  prod3 : Product  Inputs=3  OutDataType=sfix(16)  OutScaling=2^0
  prod4 : Product  OutDataType=sfix(16)  OutScaling=2^0
  sliding friction : Constant  Value=friction  OutDataType=sfix(16)  OutScaling=2^0
  velocCanon : Gain  Gain=velocCanon  ParameterDataType=sfix(16)  ParameterScaling=2^0  OutDataType=sfix(16)  OutScaling=2^0
  y inv : Gain  Gain=1./max(eps, yieldDispl)  ParameterDataType=sfix(16)  ParameterScaling=2^0  OutDataType=sfix(16)  OutScaling=2^0
  force : Outport  OutDataType=sfix(16)  OutScaling=2^0
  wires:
  integrator/1 -> prod3/2, prod3/1, prod4/1, prod1/2  "zee"
  y inv/1 -> integrator/1
  prod2/1 -> y inv/1
  Sum1/1 -> prod2/1
  prod3/1 -> Sum1/2
  one/1 -> Sum1/1
  Sum/1 -> prod3/3
  beta/1 -> Sum/1
  1-beta/1 -> Sum/2
  Sign/1 -> 1-beta/1
  prod4/1 -> Sign/1
  veloc/1 -> velocCanon/1
  prod1/1 -> force/1
  sliding friction/1 -> prod1/1
  velocCanon/1 -> prod2/2, prod4/2

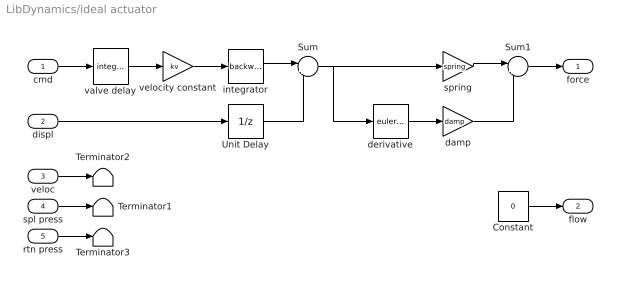
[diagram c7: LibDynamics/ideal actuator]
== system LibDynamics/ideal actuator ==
  cmd : Inport  OutDataType=sfix(16)  OutScaling=2^0
  displ : Inport  Port=2  OutDataType=sfix(16)  OutScaling=2^0
  veloc : Inport  Port=3  OutDataType=sfix(16)  OutScaling=2^0
  spl press : Inport  Port=4  OutDataType=sfix(16)  OutScaling=2^0
  rtn press : Inport  Port=5  OutDataType=sfix(16)  OutScaling=2^0
  Constant : Constant  Value=0  OutDataType=sfix(16)  OutScaling=2^0
  Sum : Sum  Inputs=|+-  OutDataType=sfix(16)  OutScaling=2^0
  Sum1 : Sum  Inputs=|++  OutDataType=sfix(16)  OutScaling=2^0
  Terminator1 : Terminator
  Terminator2 : Terminator
  Terminator3 : Terminator
  Unit Delay : UnitDelay  SampleTime=-1
  damp : Gain  Gain=damp  ParameterDataType=sfix(16)  ParameterScaling=2^0  OutDataType=sfix(16)  OutScaling=2^0
  derivative : LibDynamics/euler derivative  SystemSampleTime=-1  initialCondition=0  samplePeriod=samplePeriod
  integrator : LibDynamics/backward euler integrator  SystemSampleTime=-1  initialCondition=0  samplePeriod=samplePeriod
  spring : Gain  Gain=spring  ParameterDataType=sfix(16)  ParameterScaling=2^0  OutDataType=sfix(16)  OutScaling=2^0
  valve delay : LibDynamics/integer delay  SystemSampleTime=-1  initialCondition=0.0  sampleTime=-1  delay=round(delay/samplePeriod)
  velocity constant : Gain  Gain=kv  ParameterDataType=sfix(16)  ParameterScaling=2^0  OutDataType=sfix(16)  OutScaling=2^0
  force : Outport  OutDataType=sfix(16)  OutScaling=2^0
  flow : Outport  Port=2  OutDataType=sfix(16)  OutScaling=2^0
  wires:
  Sum1/1 -> force/1
  damp/1 -> Sum1/2
  spring/1 -> Sum1/1
  velocity constant/1 -> integrator/1
  integrator/1 -> Sum/1
  displ/1 -> Unit Delay/1
  Unit Delay/1 -> Sum/2
  Sum/1 -> spring/1, derivative/1
  derivative/1 -> damp/1
  Constant/1 -> flow/1
  cmd/1 -> valve delay/1
  veloc/1 -> Terminator2/1
  spl press/1 -> Terminator1/1
  rtn press/1 -> Terminator3/1
  valve delay/1 -> velocity constant/1

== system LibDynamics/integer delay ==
  inp : Inport  OutDataType=sfix(16)  OutScaling=2^0
  Integer Delay : simulink/Discrete/Integer Delay  vinit=initialCondition  samptime=sampleTime  NumDelays=max(delay, 1)
  Switch : Switch  Criteria=u2 ~= 0  OutDataType=sfix(16)  OutScaling=2^0
  delay > 0 : Constant  Value=delay > 0  OutDataType=sfix(16)  OutScaling=2^0
  out : Outport  OutDataType=sfix(16)  OutScaling=2^0
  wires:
  Integer Delay/1 -> Switch/1
  inp/1 -> Integer Delay/1, Switch/3
  delay > 0/1 -> Switch/2
  Switch/1 -> out/1

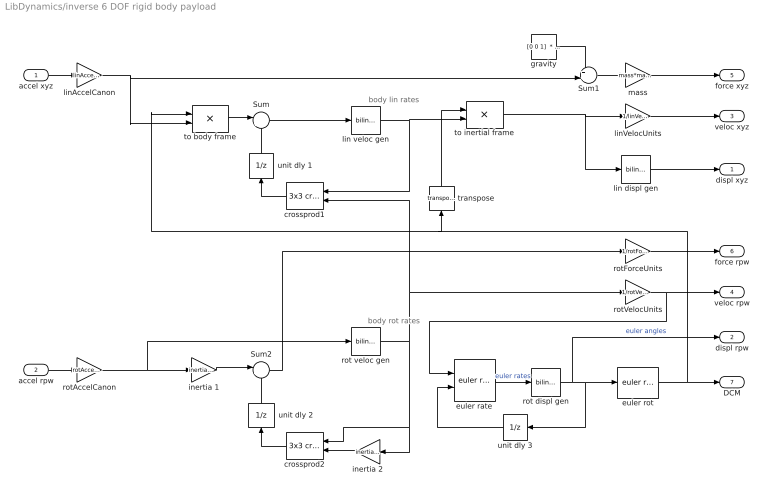
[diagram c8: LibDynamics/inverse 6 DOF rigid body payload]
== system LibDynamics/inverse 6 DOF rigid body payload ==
  note: body rot rates
  note: body lin rates
  accel xyz : Inport  OutDataType=sfix(16)  OutScaling=2^0
  accel rpw : Inport  Port=2  OutDataType=sfix(16)  OutScaling=2^0
  Sum : Sum  Inputs=|++  OutDataType=sfix(16)  OutScaling=2^0
  Sum1 : Sum  Inputs=++|  OutDataType=sfix(16)  OutScaling=2^0
  Sum2 : Sum  Inputs=|++  OutDataType=sfix(16)  OutScaling=2^0
  crossprod1 : aerospace/Axes Transformations/3x3 cross product  Orientation=left  SystemSampleTime=-1
  crossprod2 : aerospace/Axes Transformations/3x3 cross product  Orientation=left  SystemSampleTime=-1
  euler rate : LibTransforms/euler rate  SystemSampleTime=-1
  euler rot : LibTransforms/euler rot  SystemSampleTime=-1
  gravity : Constant  Value="[0 0 1]  * gee *  linAccelCanon"  OutDataType=sfix(16)  OutScaling=2^0
  inertia 1 : Gain  Gain=inertia*inertiaCanon  Multiplication=Matrix(K*u)  ParameterDataType=sfix(16)  ParameterScaling=2^0  OutDataType=sfix(16)  OutScaling=2^0
  inertia 2 : Gain  Orientation=left  Gain=inertia*inertiaCanon  Multiplication=Matrix(K*u)  ParameterDataType=sfix(16)  ParameterScaling=2^0  OutDataType=sfix(16)  OutScaling=2^0
  lin displ gen : LibDynamics/bilinear integrator  SystemSampleTime=-1  initialCondition=initialPosition(1:3)  samplePeriod=samplePeriod
  lin veloc gen : LibDynamics/bilinear integrator  SystemSampleTime=-1  initialCondition=0  samplePeriod=samplePeriod
  linAccelCanon : Gain  Gain=linAccelCanon  ParameterDataType=sfix(16)  ParameterScaling=2^0  OutDataType=sfix(16)  OutScaling=2^0
  linVelocUnits : Gain  Gain=1/linVelocCanon  ParameterDataType=sfix(16)  ParameterScaling=2^0  OutDataType=sfix(16)  OutScaling=2^0
  mass : Gain  Gain=mass*massCanon  ParameterDataType=sfix(16)  ParameterScaling=2^0  OutDataType=sfix(16)  OutScaling=2^0
  rot displ gen : LibDynamics/bilinear integrator  SystemSampleTime=-1  initialCondition=initialPosition(4:6)  samplePeriod=samplePeriod
  rot veloc gen : LibDynamics/bilinear integrator  SystemSampleTime=-1  initialCondition=0  samplePeriod=samplePeriod
  rotAccelCanon : Gain  Gain=rotAccelCanon  ParameterDataType=sfix(16)  ParameterScaling=2^0  OutDataType=sfix(16)  OutScaling=2^0
  rotForceUnits : Gain  Gain=1/rotForceCanon  ParameterDataType=sfix(16)  ParameterScaling=2^0  OutDataType=sfix(16)  OutScaling=2^0
  rotVelocUnits : Gain  Gain=1/rotVelocCanon  ParameterDataType=sfix(16)  ParameterScaling=2^0  OutDataType=sfix(16)  OutScaling=2^0
  to body frame : Product  Multiplication=Matrix(*)  OutDataType=sfix(16)  OutScaling=2^0
  to inertial frame : Product  Multiplication=Matrix(*)  OutDataType=sfix(16)  OutScaling=2^0
  transpose : Math  Orientation=up  Operator=transpose  OutDataType=sfix(16)  OutScaling=2^0
  unit dly 1 : UnitDelay  Orientation=up  SampleTime=-1
  unit dly 2 : UnitDelay  Orientation=up  SampleTime=-1
  unit dly 3 : UnitDelay  Orientation=left  X0=initialPosition(4:6)  SampleTime=-1
  displ xyz : Outport  OutDataType=sfix(16)  OutScaling=2^0
  displ rpw : Outport  Port=2  OutDataType=sfix(16)  OutScaling=2^0
  veloc xyz : Outport  Port=3  OutDataType=sfix(16)  OutScaling=2^0
  veloc rpw : Outport  Port=4  OutDataType=sfix(16)  OutScaling=2^0
  force xyz : Outport  Port=5  OutDataType=sfix(16)  OutScaling=2^0
  force rpw : Outport  Port=6  OutDataType=sfix(16)  OutScaling=2^0
  DCM : Outport  Port=7  OutDataType=sfix(16)  OutScaling=2^0
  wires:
  linAccelCanon/1 -> to body frame/2, Sum1/2
  Sum1/1 -> mass/1
  mass/1 -> force xyz/1
  accel xyz/1 -> linAccelCanon/1
  Sum2/1 -> rotForceUnits/1
  rotForceUnits/1 -> force rpw/1
  inertia 1/1 -> Sum2/1
  rotAccelCanon/1 -> inertia 1/1, rot veloc gen/1
  accel rpw/1 -> rotAccelCanon/1
  to body frame/1 -> Sum/1
  gravity/1 -> Sum1/1
  crossprod1/1 -> unit dly 1/1
  transpose/1 -> to inertial frame/1
  to inertial frame/1 -> linVelocUnits/1, lin displ gen/1
  linVelocUnits/1 -> veloc xyz/1
  inertia 2/1 -> crossprod2/2
  rotVelocUnits/1 -> veloc rpw/1, euler rate/1
  rot displ gen/1 -> displ rpw/1, unit dly 3/1, euler rot/1  "euler angles"
  crossprod2/1 -> unit dly 2/1
  Sum/1 -> lin veloc gen/1
  lin displ gen/1 -> displ xyz/1
  euler rot/1 -> DCM/1, transpose/1, to body frame/1
  euler rate/1 -> rot displ gen/1  "euler rates"
  lin veloc gen/1 -> crossprod1/1, to inertial frame/2
  rot veloc gen/1 -> inertia 2/1, crossprod2/1, rotVelocUnits/1, crossprod1/2
  unit dly 1/1 -> Sum/2
  unit dly 2/1 -> Sum2/2
  unit dly 3/1 -> euler rate/2
